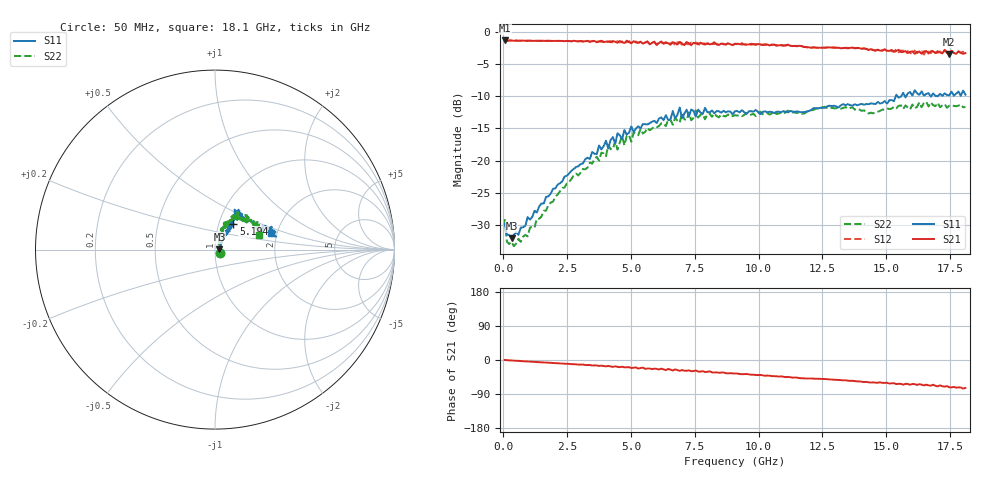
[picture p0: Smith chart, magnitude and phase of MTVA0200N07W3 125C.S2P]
! Network Analyzer HP8720D.06.14 Serial No. US36140669
!  7 Jul 2005  07:49:17
! Frequency  S11  S21  S12  S22
# HZ  S  DB R 50
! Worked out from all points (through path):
!   201 points, 50 MHz to 18.1 GHz, reference 50 ohm
!   highest |S21| = -1.36 dB at 50 MHz (marker M1); lowest = -3.5 dB at 17.47 GHz (marker M2)
!   group delay of S21, straight-line fit = 11.3 ps
!   lowest |S11| = -32.1 dB at 320.8 MHz (marker M3), VSWR 1.05, Z = 52.5 + j0.268 ohm
!   |S11| at or under -10 dB: start of sweep to 15.37 GHz; 15.44 GHz to 15.59 GHz (148.4 MHz wide, 0.957 % of centre); 15.7277 GHz to 15.78272 GHz (55.02 MHz wide, 0.349 % of centre)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
!   |S22| runs from -33.3 to -10.9 dB; largest |S21 - S12| = 0.05
!   S11 on the Smith chart (normalised r, x): 50 MHz: 1.06, -0.03; 5.194 GHz: 1.17, +0.35; 18.1 GHz: 1.86, +0.38
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5e7  -29.80 -30.3  -1.36 0.1  -1.37 0.2  -29.08 -30.5
1.4025e8  -31.50 -14.0  -1.43 -0.4  -1.41 -0.4  -32.60 -14.8
3.2075e8  -32.08 5.9  -1.36 -1.0  -1.38 -1.1  -32.62 4.0
9.525e8  -28.78 32.9  -1.42 -3.9  -1.38 -3.9  -31.78 40.4
3.1185e9  -20.46 54.7  -1.51 -12.0  -1.53 -12.4  -21.32 70.4
4.021e9  -16.92 57.0  -1.53 -16.9  -1.54 -15.7  -19.33 67.9
4.11125e9  -18.13 57.5  -1.50 -15.5  -1.60 -17.0  -17.59 68.0
4.47225e9  -15.76 53.4  -1.72 -18.0  -1.49 -17.1  -18.31 72.7
5.19425e9  -15.03 54.5  -1.68 -19.6  -1.50 -20.1  -15.89 70.7
6.09675e9  -13.48 57.0  -1.75 -25.0  -1.62 -24.5  -14.66 62.1
6.7285e9  -13.49 62.9  -1.75 -24.8  -2.08 -25.6  -13.38 56.7
6.909e9  -11.76 59.5  -1.58 -28.5  -1.65 -26.3  -14.12 57.6
6.99925e9  -13.43 59.2  -1.80 -26.5  -2.03 -28.9  -12.65 57.5
7.36025e9  -12.09 53.7  -2.10 -29.6  -1.69 -28.6  -13.74 60.7
7.54075e9  -13.18 56.5  -1.82 -27.6  -1.69 -31.0  -12.21 59.1
7.90175e9  -11.83 58.0  -2.00 -31.8  -1.84 -29.9  -13.60 55.1
9.075e9  -12.33 55.7  -1.89 -35.6  -1.86 -35.7  -12.96 49.2
1.21435e10  -11.89 40.1  -2.45 -49.0  -2.38 -49.0  -12.13 49.4
1.512175e10  -10.64 22.2  -2.98 -62.2  -2.74 -61.8  -11.98 39.5
1.61145e10  -9.08 16.1  -3.42 -63.8  -2.92 -64.2  -11.91 35.1
1.746825e10  -9.89 14.6  -3.46 -71.9  -3.46 -71.9  -11.49 23.9
1.81e10  -9.76 16.3  -3.33 -73.7  -3.58 -73.4  -11.68 18.2
